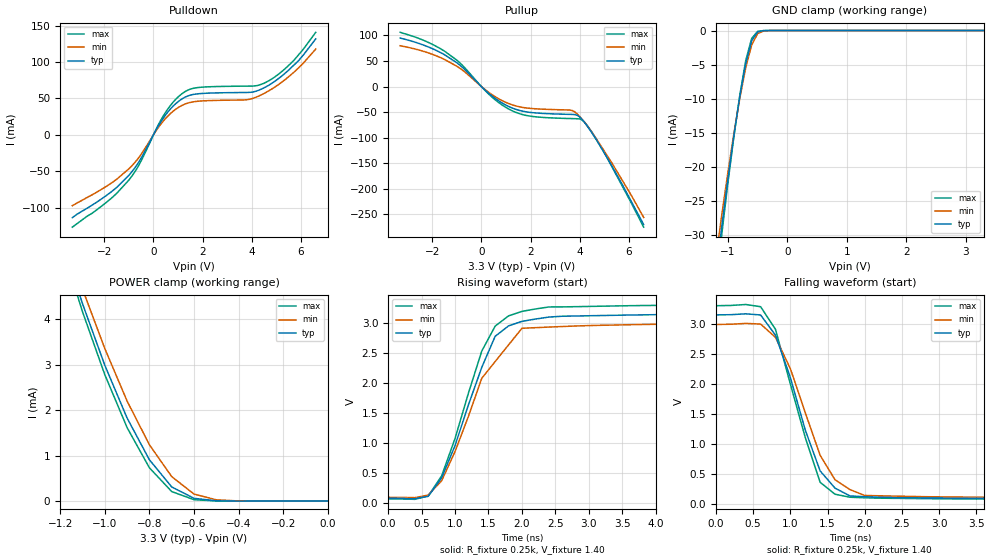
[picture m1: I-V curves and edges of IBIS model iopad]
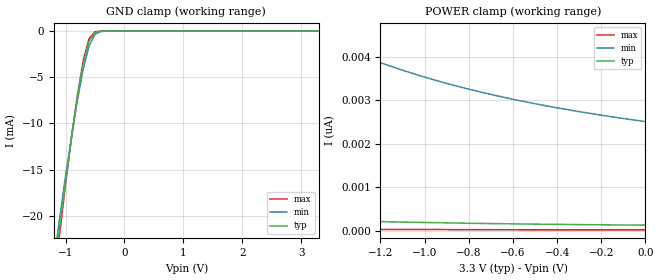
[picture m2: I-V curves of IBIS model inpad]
| IBIS file 70v3389.ibs created by s2ibis2 version 1.1
| North Carolina State University Electronics Research Laboratory  1995
[IBIS ver]   2.1
[File name]   70v3389.ibs
[File Rev]   1.0
[Date]   12/16/98 mff
[Source]   Integrated Device Technology, Inc.
[Notes]   1.Temperatures: typ=25C, min=70C, max=0C 2.RRmp rates based on
   50 ohm load.
[Disclaimer] Integrated Device Technology, Inc. ("IDT") hereby grants the
   user of this IBIS model a non-exclusive, nontransferable
   license to use this IBIS model under the following terms. The
   user is granted this license only to use the IBIS model and is
   not granted rights to sell, copy (except as needed to run the
   IBIS model), rent, lease or sub-license the IBIS model in
   whole or in part, or in modified form to anyone. The User may
   modify the IBIS model to suit its specific applications, but
   rights to derivative works and such modifications shall belong
   to IDT. This IBIS model is provided on an AS IS" basis and IDT
   makes absolutely no warranty with respect to the information
   contained herein. IDT DISCLAIMS AND CUSTOMER WAIVES ALL
   WARRANTIES, EXPRESS AND IMPLIED, INCLUDING WARRANTIES OF
   MERCHANTABILITY AND FITNESS FOR A PARTICULAR PURPOSE. THE
   ENTIRE RISK AS TO QUALITY AND PERFORMANCE IS WITH THE USER
   ACCORDINGLY, IN NO EVENT SHALL IDT BE LIABLE FOR ANY DIRECT OR
   INDIRECT DAMAGES, WHETHER IN CONTRACT OR TORT, INCLUDING ANY
   LOST PROFITS OR OTHER INCIDENTAL, CONSEQUENTIAL, EXEMPLARY, OR
   PUNITIVE DAMAGES ARISING OUT OF THE USE OR APPLICATION OF THE
   IBIS model. Further, IDT reserves the right to make changes
   without notice to any product herein to improve reliability,
   function, or design. IDT does not convey any license under
   patent rights or any other intellectual property rights,
   including those of third parties. IDT is not obligated to
   provide maintenance or support for the licensed IBIS model.
[Copyright]   Copyright 1998, Integrated Device Technology, Inc. all rights
   reserved
|   Component 70v3389pk128
[Component]   70v3389pk128
[Manufacturer]   Integrated Device Technology
[Package]
| variable   typ   min   max
R_pkg   100.00m   50.00m   0.30
L_pkg   4.70nH   3.20nH   6.70nH
C_pkg   1.00pF   0.15pF   2.90pF
[Pin]  signal_name   model_name   R_pin   L_pin   C_pin
5   io9l   iopad
6   io9r   iopad
7   vddql   POWER
8   vss   GND
9   io10l   iopad
10   io10r   iopad
11   vddqr   POWER
12   vss   GND
13   io11l   iopad
14   io11r   iopad
15   io12l   iopad
16   io12r   iopad
17   vdd   POWER
18   vdd   POWER
19   vss   GND
20   vss   GND
21   io13r   iopad
22   io13l   iopad
23   io14r   iopad
24   io14l   iopad
25   io15r   iopad
26   io15l   iopad
27   vddql   POWER
28   vss   GND
29   io16r   iopad
30   io16l   iopad
31   vddqr   POWER
32   vss   GND
33   io17r   iopad
34   io17l   iopad
37   a15r   inpad
38   a14r   inpad
39   a13r   inpad
40   a12r   inpad
41   a11r   inpad
42   a10r   inpad
43   a9r   inpad
44   a8r   inpad
45   a7r   inpad
46   ubr#   inpad
47   lbr#   inpad
48   ce1r   inpad
49   ce0r   inpad
50   vdd   POWER
51   vdd   POWER
52   vss   GND
53   vss   GND
54   clkr   inpad
55   oer#   inpad
56   rwr#   inpad
57   adsr#   inpad
58   cntenr#   inpad
59   cntrstr#   inpad
60   a6r   inpad
61   a5r   inpad
62   a4r   inpad
63   a3r   inpad
64   a2r   inpad
65   a1r   inpad
66   a0r   inpad
67   vdd   POWER
68   io0l   iopad
69   io0r   iopad
70   vddqr   POWER
71   vss   GND
72   io1l   iopad
73   io1r   iopad
74   vddql   POWER
75   vss   GND
76   io2l   iopad
77   io2r   iopad
78   io3l   iopad
79   io3r   iopad
80   io4l   iopad
81   io4r   iopad
82   vss   GND
83   vss   GND
84   vdd   POWER
85   vdd   POWER
86   io5r   iopad
87   io5l   iopad
88   io6r   iopad
89   io6l   iopad
90   vddqr   POWER
91   vss   GND
92   io7r   iopad
93   io7l   iopad
94   vddql   POWER
95   vss   GND
97   io8r   iopad
98   io8l   iopad
100   vdd   POWER
101   a0l   inpad
102   a1l   inpad
103   a2l   inpad
104   a3l   inpad
105   a4l   inpad
106   a5l   inpad
107   a6l   inpad
108   cntrstl#   inpad
109   cntenl#   inpad
110   adsl#   inpad
111   rwl#   inpad
112   oel#   inpad
113   clkl   inpad
114   vss   GND
115   vss   GND
116   vdd   POWER
117   vdd   POWER
118   ce0l   inpad
119   ce1l   inpad
120   lbl#   inpad
121   ubl#   inpad
122   a7l   inpad
123   a8l   inpad
124   a9l   inpad
125   a10l   inpad
126   a11l   inpad
127   a12l   inpad
128   a13l   inpad
1   a14l   inpad
2   a15l   inpad
3   vss   GND
| in   in   dummy_model
| oe   oe   dummy_model
[Pin Mapping]  pulldown_ref   pullup_ref   gnd_clamp_ref   power_clamp_ref
5   vss   vddql
6   vss   vddqr
7   NC   vddql
8   vss   NC
9   vss   vddql
10   vss   vddqr
11   NC   vddqr
12   vss   NC
13   vss   vddql
14   vss   vddqr
15   vss   vddql
16   vss   vddqr
17   NC   vdd
18   NC   vdd
19   vss   NC
20   vss   NC
21   vss   vddqr
22   vss   vddql
23   vss   vddqr
24   vss   vddql
25   vss   vddqr
26   vss   vddql
27   NC   vddql
28   vss   NC
29   vss   vddqr
30   vss   vddql
31   NC   vddqr
32   vss   NC
33   vss   vddqr
34   vss   vddql
37   vss   vdd
38   vss   vdd
39   vss   vdd
40   vss   vdd
41   vss   vdd
42   vss   vdd
43   vss   vdd
44   vss   vdd
45   vss   vdd
46   vss   vdd
47   vss   vdd
48   vss   vdd
49   vss   vdd
50   NC   vdd
51   NC   vdd
52   vss   NC
53   vss   NC
54   vss   vdd
55   vss   vdd
56   vss   vdd
57   vss   vdd
58   vss   vdd
59   vss   vdd
60   vss   vdd
61   vss   vdd
62   vss   vdd
63   vss   vdd
64   vss   vdd
65   vss   vdd
66   vss   vdd
67   NC   vdd
68   vss   vddql
69   vss   vddqr
70   NC   vddqr
71   vss   NC
72   vss   vddql
73   vss   vddqr
74   NC   vddql
75   vss   NC
76   vss   vddql
77   vss   vddqr
78   vss   vddql
79   vss   vddqr
80   vss   vddql
81   vss   vddqr
82   vss   NC
83   vss   NC
84   NC   vdd
85   NC   vdd
86   vss   vddqr
87   vss   vddql
88   vss   vddqr
89   vss   vddql
90   NC   vddqr
91   vss   NC
92   vss   vddqr
93   vss   vddql
94   NC   vddql
95   vss   NC
97   vss   vddqr
98   vss   vddql
100   NC   vdd
101   vss   vdd
102   vss   vdd
103   vss   vdd
104   vss   vdd
105   vss   vdd
106   vss   vdd
107   vss   vdd
108   vss   vdd
109   vss   vdd
110   vss   vdd
111   vss   vdd
112   vss   vdd
113   vss   vdd
114   vss   NC
115   vss   NC
116   NC   vdd
117   NC   vdd
118   vss   vdd
119   vss   vdd
120   vss   vdd
121   vss   vdd
122   vss   vdd
123   vss   vdd
124   vss   vdd
125   vss   vdd
126   vss   vdd
127   vss   vdd
128   vss   vdd
1   vss   vdd
2   vss   vdd
3   vss   NC
| Models and submodels in the file (2): iopad (I/O), inpad (Input)
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|in   NC   NC
|oe   NC   NC
|   Model iopad
[Model]   iopad
Model_type   I/O
Polarity   Non-Inverting
Enable   Active-High
Vinl =  0.800V
Vinh =  2.000V
Vmeas =  1.500V
C_comp   1.00pF   NA   NA
[Temperature Range]   25.00   70.00   0.000
[Voltage Range]   3.30V   3.15V   3.45V
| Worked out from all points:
|   slope of the pulldown table from 0 to 0.495 V, typ, clamps not added: 18 ohm
|   slope of the pullup table from 0 to 0.495 V, typ, clamps not added: 23.7 ohm
|   GND clamp passes 1 mA (typ) near -0.56 V on its own axis
|   POWER clamp passes 1 mA (typ) near -0.81 V on its own axis
|   rising waveform, R_fixture 0.25k, V_fixture 1.40: 20-80 % time 605ps typ, 716ps min, 576ps max; typ from 0.082 V to 3.15 V
|   falling waveform, R_fixture 0.25k, V_fixture 1.40: 20-80 % time 479ps typ, 525ps min, 448ps max; typ from 3.15 V to 0.082 V
[Pulldown]
| voltage   I(typ)   I(min)   I(max)
-3.3V     -114mA     -97.5mA    -127mA
-1.9V     -83.06mA   -70.53mA   -92.53mA
-1V       -55.69mA   -46.78mA   -62.24mA
-600mV    -37.64mA   -31.5mA    -42.12mA
400mV     22.98mA    18.97mA    26.02mA
1.1V      48.05mA    39.4mA     54.97mA
1.8V      56.39mA    46.16mA    65mA
3.8V      58.27mA    48.27mA    67mA
4.5V      64.64mA    56.89mA    71.01mA
5.1V      77.7mA     69.5mA     83.74mA
5.7V      95.54mA    85.76mA    102mA
6.6V      132mA      118mA      141mA
[Pullup]
| voltage   I(typ)   I(min)   I(max)
-3.3V     94.72mA    79.74mA    106mA
-2.3V     80.13mA    68mA       89.32mA
-1.5V     62.22mA    52.99mA    69.19mA
-800mV    38.7mA     33.19mA    42.88mA
400mV     -17.28mA   -14.82mA   -19.29mA
1.2V      -40.94mA   -34.88mA   -46.19mA
2V        -50.67mA   -42.77mA   -58.01mA
3.6V      -54.45mA   -46.05mA   -62.6mA
4V        -59.66mA   -58.71mA   -63.48mA
4.3V      -76.87mA   -76.45mA   -75.79mA
4.9V      -122mA     -119mA     -121mA
6.6V      -270mA     -256mA     -275mA
[GND_clamp]
| voltage   I(typ)   I(min)   I(max)
-3.3V     -213mA     -195mA     -224mA
-1.2V     -35.67mA   -33.21mA   -37.24mA
-1.1V     -28.54mA   -26.85mA   -29.61mA
-1V       -21.76mA   -20.81mA   -22.35mA
-900mV    -15.43mA   -15.14mA   -15.59mA
-800mV    -9.676mA   -9.946mA   -9.478mA
-700mV    -4.805mA   -5.441mA   -4.393mA
-600mV    -1.485mA   -2.103mA   -1.146mA
-500mV    -215uA     -458uA     -124uA
-400mV    -17.97uA   -58.09uA   -7.861uA
-300mV    -1.106uA   -5.62uA    -349nA
3.3V      143pA      13.86nA    17.08pA
[POWER_clamp]
| voltage   I(typ)   I(min)   I(max)
-3.3V     54.48mA    50.56mA    57.22mA
-1.2V     5.852mA    6.099mA    5.729mA
-1.1V     4.338mA    4.66mA     4.161mA
-1V       2.985mA    3.352mA    2.778mA
-900mV    1.825mA    2.198mA    1.615mA
-800mV    908uA      1.238mA    732uA
-700mV    312uA      538uA      210uA
-600mV    61.42uA    155uA      31.29uA
-500mV    7.539uA    28.27uA    3.013uA
-400mV    726nA      3.93uA     220nA
0V        143pA      2.833nA    18.39pA
[Ramp]
| variable   typ   min   max
dV/dt_r   1.24/1.42n   1.10/1.61n   1.37/1.50n
dV/dt_f   1.37/1.27n   1.20/1.54n   1.50/1.16n
R_load = 50.00
[Rising Waveform]
R_fixture = 0.25k
V_fixture = 1.40
| time   V(typ)   V(min)   V(max)
0s        81.93mV    98.35mV    72.87mV
600ps     115mV      136mV      121mV
800ps     421mV      373mV      454mV
1ns       956mV      858mV      1.074V
1.4ns     2.258V     2.076V     2.528V
1.6ns     2.773V     2.353V     2.942V
1.8ns     2.946V     2.63V      3.112V
2ns       3.021V     2.906V     3.187V
2.4ns     3.092V     2.926V     3.26V
19.8ns    3.148V     2.988V     3.301V
[Falling Waveform]
R_fixture = 0.25k
V_fixture = 1.40
| time   V(typ)   V(min)   V(max)
0s        3.148V     2.988V     3.301V
600ps     3.146V     2.995V     3.284V
800ps     2.81V      2.773V     2.907V
1ns       2.103V     2.251V     1.994V
1.2ns     1.229V     1.519V     1.105V
1.4ns     547mV      807mV      358mV
1.6ns     260mV      400mV      158mV
1.8ns     130mV      236mV      108mV
3.8ns     87.38mV    105mV      76.98mV
19.8ns    81.93mV    98.32mV    72.85mV
|   Model inpad
[Model]   inpad
Model_type   Input
Vinl =  0.800V
Vinh =  2.000V
C_comp   1.00pF   NA   NA
[Temperature Range]   25.00   70.00   0.000
[Voltage Range]   3.30V   3.15V   3.45V
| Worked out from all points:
|   GND clamp passes 1 mA (typ) near -0.59 V on its own axis
[GND_clamp]
| voltage   I(typ)   I(min)   I(max)
-3.3V     -151mA     -139mA     -158mA
-1.2V     -26.48mA   -24.89mA   -27.46mA
-1.1V     -21.24mA   -20.19mA   -21.89mA
-1V       -16.24mA   -15.68mA   -16.56mA
-900mV    -11.52mA   -11.43mA   -11.55mA
-800mV    -7.21mA    -7.515mA   -6.992mA
-700mV    -3.543mA   -4.098mA   -3.185mA
-600mV    -1.064mA   -1.569mA   -793uA
-500mV    -149uA     -338uA     -82.26uA
-400mV    -12.54uA   -43.03uA   -5.213uA
-300mV    -780nA     -4.214uA   -234nA
3.3V      126pA      2.619nA    15.18pA
[POWER_clamp]
| voltage   I(typ)   I(min)   I(max)
-3.3V     884pA      14.8nA     129pA
-2.9V     654pA      11.11nA    94.51pA
-2.5V     486pA      8.384nA    69.46pA
-2V       340pA      6.023nA    47.82pA
-1.6V     262pA      4.75nA     36.18pA
-1.5V     247pA      4.498nA    33.87pA
-1.4V     232pA      4.268nA    31.77pA
-1.2V     208pA      3.867nA    28.12pA
-1V       188pA      3.534nA    25.09pA
-800mV    170pA      3.257nA    22.58pA
-400mV    144pA      2.827nA    18.74pA
0V        126pA      2.51nA     16.01pA
